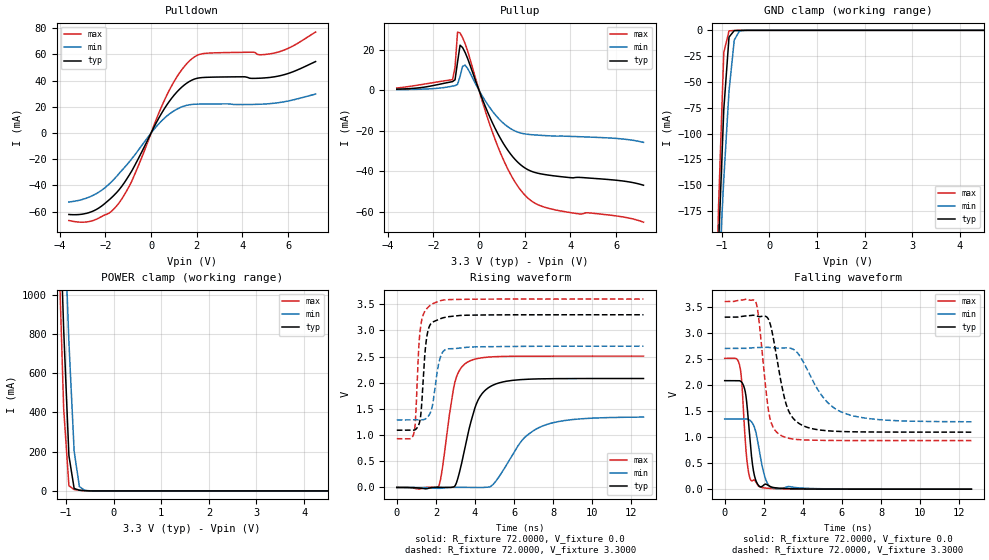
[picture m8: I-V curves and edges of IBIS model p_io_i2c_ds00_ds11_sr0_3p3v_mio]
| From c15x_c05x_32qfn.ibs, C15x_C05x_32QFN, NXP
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[Model] p_io_i2c_ds00_ds11_sr0_3p3v_mio
|   Model p_io_i2c_ds00_ds11_sr0_3p3v_mio
| This model was characterised for following simulation conditions:
| External (pad) voltage:
|   - Typ: 3.3V,   - Min: 2.7V,   - Max: 3.6V
| Library cells for typ/min/max conditions are connected as defined below:
|  pad - External Pad
|  ipp_do_lv - Core Input
|  ipp_obe_lv - Output Buffer Enable
|  IOGC - NC
|  REFH3V3 - REFH3V3
|  REFL3V3 - REFL3V3
|  ZI - NC
|  abut_ncal_vddio[1] - vddio
|  abut_ncal_vddio[2] - vddio
|  abut_ncal_vddio[3] - vssio
|  abut_ncal_vddio[4] - vddio
|  abut_ncal_vddio[5] - vddio
|  abut_ncal_vddio[6] - vssio
|  abut_pcal_vddio[1] - vssio
|  abut_pcal_vddio[2] - vssio
|  abut_pcal_vddio[3] - vddio
|  abut_pcal_vddio[4] - vssio
|  abut_pcal_vddio[5] - vssio
|  abut_pcal_vddio[6] - vddio
|  ipp_do_1p8v - ipp_do_1p8v
|  ipp_dse_lv[0] - 0
|  ipp_dse_lv[1] - vdd_lv
|  ipp_eftd_lv - NC
|  ipp_ina_mux_vddio - NC
|  ipp_ina_mux_vddio[0] - NC
|  ipp_ina_mux_vddio[1] - NC
|  ipp_ina_r0_vddio - NC
|  ipp_ina_r0a_vddio - NC
|  ipp_ina_r0b_vddio - NC
|  ipp_ina_r0c_vddio - NC
|  ipp_ina_r0d_vddio - NC
|  ipp_ina_r0e_vddio - NC
|  ipp_ina_r0f_vddio - NC
|  ipp_ina_r300_vddio - NC
|  ipp_ina_r300a_vddio - NC
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Model_type I/O
Polarity   Non-Inverting
Enable   Active-High
Vinl =   0.9900V
Vinh =   2.3100V
Vmeas =  1.6500V
Cref =   30.0000pF
Rref =   1.0000M
Vref =   3.3000V
C_comp   1.4149pF   1.3702pF   1.4746pF
|C_comp_pullup   0.5853pF   0.6306pF   0.5566pF
|C_comp_pulldown   0.7311pF   0.7416pF   0.7172pF
[Model Spec]
| variable   typ   min   max
Vinh   2.3100V   1.8900V   2.5200V
Vinl   0.9900V   0.8100V   1.0800V
[Temperature Range]   25.0000   0.1250k   -40.0000
[Voltage Range]   3.3000V   2.7000V   3.6000V
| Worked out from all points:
|   slope of the pulldown table from 0 to 0.495 V, typ, clamps not added: 30.7 ohm
|   slope of the pullup table from 0 to 0.495 V, typ, clamps not added: 35.9 ohm
|   GND clamp passes 1 mA (typ) near -0.75 V on its own axis
|   POWER clamp passes 1 mA (typ) near -0.57 V on its own axis
|   rising waveform, R_fixture 72.0000, V_fixture 0.0: 20-80 % time 863ps typ, 1.61ns min, 587ps max; typ from 0 V to 2.08 V
|   rising waveform, R_fixture 72.0000, V_fixture 3.3000: 20-80 % time 264ps typ, 349ps min, 235ps max; typ from 1.09 V to 3.3 V
|   falling waveform, R_fixture 72.0000, V_fixture 0.0: 20-80 % time 317ps typ, 426ps min, 270ps max; typ from 2.08 V to 0 V
|   falling waveform, R_fixture 72.0000, V_fixture 3.3000: 20-80 % time 724ps typ, 1.48ns min, 457ps max; typ from 3.3 V to 1.09 V
[Pulldown]
|Voltage   I(typ)   I(min)   I(max)
-3.6V     -62.23mA   -52.7mA    -66.82mA
-2.5V     -59.31mA   -47.25mA   -66.6mA
-1.84V    -51.07mA   -39.04mA   -61.22mA
-1.4V     -43.29mA   -30.9mA    -53.3mA
-850mV    -29.1mA    -19.8mA    -36.9mA
140mV     4.939mA    3.095mA    6.557mA
800mV     24.23mA    14.5mA     32.79mA
1.35V     35.15mA    20.01mA    48.49mA
1.79V     40.41mA    21.82mA    56.77mA
2.45V     42.54mA    22.16mA    60.95mA
5.42V     42.98mA    22.81mA    61.18mA
7.2V      54.57mA    29.73mA    77.07mA
[Pullup]
|Voltage   I(typ)   I(min)   I(max)
-3.6V     528.7uA    283.5uA    1.096mA
-1.16V    4.253mA    2.05mA     5.214mA
-1.05V    5.16mA     2.299mA    11.28mA
-940mV    13.88mA    2.903mA    28.69mA
-830mV    22.22mA    6.81mA     28.28mA
-720mV    21.08mA    11.76mA    25.94mA
-610mV    18.66mA    12.39mA    23.05mA
820mV     -21.34mA   -13.5mA    -27.66mA
1.48V     -32.86mA   -19.56mA   -43.47mA
2.03V     -38.49mA   -21.57mA   -52mA
3.24V     -42.16mA   -22.57mA   -58.77mA
7.2V      -46.85mA   -25.7mA    -65.08mA
[GND_clamp]
|Voltage   I(typ)   I(min)   I(max)
-3.6V     -4.327A    -3.181A    -5.901A
-1.18V    -358.9mA   -350.6mA   -379.3mA
-1.07V    -208.2mA   -244.2mA   -170.8mA
-960mV    -76.59mA   -144.3mA   -21.58mA
-850mV    -6.561mA   -58.74mA   -508.1uA
-740mV    -273.3uA   -9.382mA   -183.5uA
-630mV    -73.8uA    -593.1uA   -76.7uA
-410mV    -3.432uA   -9.016uA   -2.096uA
7.2V      0A         0A         0A
[POWER_clamp]
|Voltage   I(typ)   I(min)   I(max)
-3.6V     20.44A     18.76A     22.48A
-1.16V    1.647A     2.216A     1.289A
-1.05V    823.6mA    1.482A     419.2mA
-940mV    180.4mA    758.9mA    26.72mA
-830mV    12.56mA    202.9mA    6.794mA
-720mV    3.422mA    22.23mA    3.58mA
-610mV    1.373mA    2.923mA    1.344mA
7.2V      0A         0A         0A
[Ramp]
| variable   typ   min   max
dV/dt_r  1.2490/0.8627n   0.8067/1.6135n   1.5058/0.5871n
dV/dt_f  1.3237/0.7240n   0.8444/1.4823n   1.6011/0.4566n
R_load = 72.0000
[Rising Waveform]
R_fixture= 72.0000
V_fixture= 0.0
V_fixture_min= 0.0
V_fixture_max= 0.0
|time   V(typ)   V(min)   V(max)
0s        1.645nV    121.1nV    5.564nV
2.146ns   2.962mV    -17.6mV    26.34mV
2.318ns   2.071mV    -13.03mV   327.5mV
2.976ns   29.54mV    1.609mV    2.014V
3.67ns    1.071V     752.5uV    2.406V
4.261ns   1.738V     -1.654mV   2.473V
5.199ns   1.994V     187.2mV    2.502V
6.44ns    2.063V     914mV      2.509V
7.456ns   2.076V     1.174V     2.509V
12.62ns   2.082V     1.345V     2.51V
[Rising Waveform]
R_fixture= 72.0000
V_fixture= 3.3000
V_fixture_min= 2.7000
V_fixture_max= 3.6000
|time   V(typ)   V(min)   V(max)
0s        1.093V     1.29V      931.4mV
882.8ps   1.095V     1.29V      1.047V
964.2ps   1.109V     1.29V      1.337V
1.145ns   1.219V     1.29V      2.792V
1.25ns    1.474V     1.29V      3.147V
1.516ns   2.831V     1.323V     3.408V
1.836ns   3.159V     1.589V     3.51V
2.195ns   3.219V     2.446V     3.564V
2.546ns   3.257V     2.643V     3.588V
12.62ns   3.3V       2.7V       3.6V
[Falling Waveform]
R_fixture= 72.0000
V_fixture= 0.0
V_fixture_min= 0.0
V_fixture_max= 0.0
|time   V(typ)   V(min)   V(max)
0s        2.082V     1.348V     2.51V
739.5ps   2.082V     1.348V     2.41V
860.7ps   2.055V     1.348V     2.113V
993.8ps   1.955V     1.349V     1.276V
1.254ns   1.1V       1.331V     262mV
1.485ns   323mV      1.22V      176.9mV
1.784ns   52.42mV    708.9mV    45.75mV
2.131ns   92.35mV    154.4mV    19.06mV
2.554ns   28.15mV    15.59mV    9.812mV
12.62ns   4.207uV    42.51uV    732.7nV
[Falling Waveform]
R_fixture= 72.0000
V_fixture= 3.3000
V_fixture_min= 2.7000
V_fixture_max= 3.6000
|time   V(typ)   V(min)   V(max)
0s        3.3V       2.7V       3.6V
1.595ns   3.326V     2.716V     3.586V
1.743ns   3.311V     2.719V     3.273V
2.271ns   3.233V     2.719V     1.441V
2.883ns   2.053V     2.704V     1.03V
3.231ns   1.534V     2.71V      980.5mV
3.726ns   1.28V      2.614V     952.2mV
5.033ns   1.127V     1.762V     935.2mV
6.102ns   1.104V     1.46V      932.9mV
12.62ns   1.094V     1.293V     931.5mV
